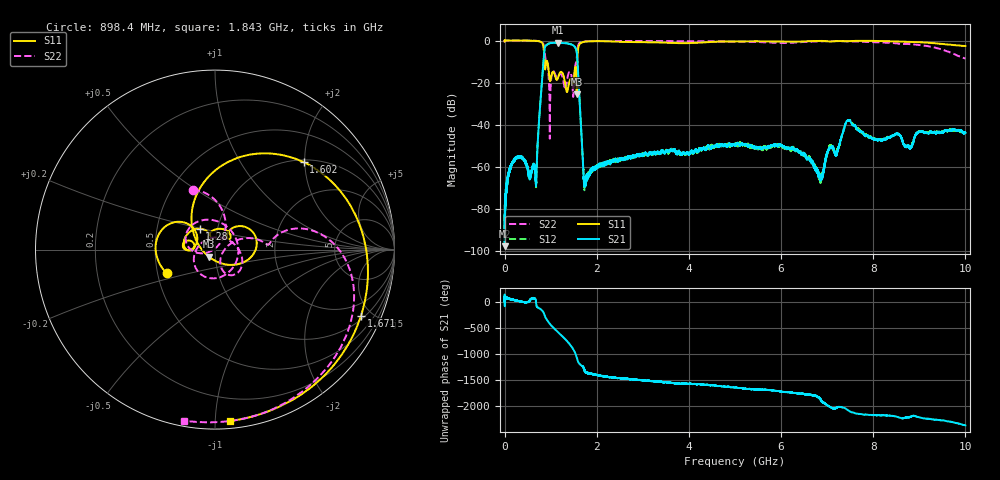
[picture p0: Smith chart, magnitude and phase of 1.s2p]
!Keysight Technologies,N5232A,MY52221221,A.10.65.11
!Date: Friday, October 13, 2023 15:51:17
!Correction: S11(Full 2 Port(1,4))
!S41(Full 2 Port(1,4))
!S14(Full 2 Port(1,4))
!S44(Full 2 Port(1,4))
!S2P File: Measurements: S11, S41, S14, S44:
# Hz S  RI  R 50
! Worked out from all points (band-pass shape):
!   16001 points, 300 kHz to 10 GHz, reference 50 ohm
!   highest |S21| = -1.04 dB at 1.157 GHz (marker M1); lowest = -97.8 dB at 3.425 MHz (marker M2)
!   |S21| within 3 dB of the highest: 868.3 MHz to 1.551 GHz (682.8 MHz wide, 56.4 % of centre)
!   lowest |S11| = -25.7 dB at 1.565 GHz (marker M3), VSWR 1.11, Z = 46.5 - j3.66 ohm
!   |S11| at or under -10 dB: 867.6 MHz to 902.7 MHz (35.09 MHz wide, 3.96 % of centre); 925.2 MHz to 1.577 GHz (652.2 MHz wide, 52.1 % of centre)
!   |S22| runs from -46.7 to 0.0 dB; largest |S21 - S12| = 0.012
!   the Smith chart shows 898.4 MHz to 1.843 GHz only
!   S11 on the Smith chart (normalised r, x): 898.4 MHz: 0.56, -0.16; 1.28 GHz: 0.82, +0.20; 1.602 GHz: 1.05, +1.98; 1.671 GHz: 1.19, -4.33; 1.843 GHz: 0.05, -1.09
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300000  1.003 -0.00511  7.06e-05 2.1e-05  0.000125 1.97e-05  1.003 -0.00631
3424906  1.001 -0.0126  2.96e-06 -1.26e-05  2.47e-05 8.22e-05  1 -0.0132
2.240433e8  0.6449 -0.7613  0.00115 0.000946  0.00114 0.001  0.6518 -0.7578
6.602802e8  -0.8699 -0.4649  0.000336 0.000764  0.000366 0.000824  -0.8325 -0.5291
8.084008e8  -0.6578 0.6066  -0.087 -0.0428  -0.0867 -0.0436  -0.8379 0.3967
8.983981e8  -0.2693 -0.1322  0.4947 0.5838  0.4967 0.5795  -0.1234 0.3328
1.020269e9  -0.1569 -0.00294  -0.0854 -0.8677  -0.0853 -0.8676  -0.1467 0.0123
1.15714e9  -0.1277 -0.00264  -0.7247 0.511  -0.7179 0.5078  0.1231 -0.0546
1.279637e9  -0.0862 0.1164  0.6442 0.5831  0.6439 0.5848  -0.1005 0.00634
1.407133e9  -0.0145 0.1043  0.1349 -0.8187  0.1343 -0.817  0.1405 -0.1126
1.479006e9  0.0797 0.0578  -0.7684 -0.1495  -0.7695 -0.1489  0.0297 -0.058
1.564628e9  -0.0344 -0.0392  0.5057 0.2033  0.5021 0.2065  0.3527 0.0849
1.602127e9  0.4941 0.4872  0.0298 -0.1178  0.031 -0.1204  0.7736 -0.2231
1.667125e9  0.8258 -0.3264  -0.00453 -0.00391  -0.00455 -0.00419  0.5105 -0.7713
1.6715e9  0.814 -0.3673  -0.00384 -0.00298  -0.00396 -0.00326  0.4881 -0.7891
1.842745e9  0.0818 -0.9549  0.000176 0.000606  0.000182 0.000719  -0.1704 -0.9534
3.33395e9  -0.8736 0.2235  4.65e-05 -0.00218  0.000109 -0.00221  -0.9556 0.1648
5.00015e9  -0.5495 0.7845  -0.00303 0.0011  -0.00333 0.00119  -0.5707 0.7535
6.666975e9  0.0254 0.9703  0.00137 0.000308  0.00122 0.000306  -0.0417 0.9417
7.456326e9  0.2999 0.912  0.00229 0.0124  0.00219 0.012  0.3496 0.8872
8.3338e9  0.6329 0.7242  0.00465 -0.00177  0.00472 -0.00176  0.6834 0.567
1e10  0.7146 -0.1915  -0.00552 0.00324  -0.00544 0.00335  -0.2588 -0.2718
